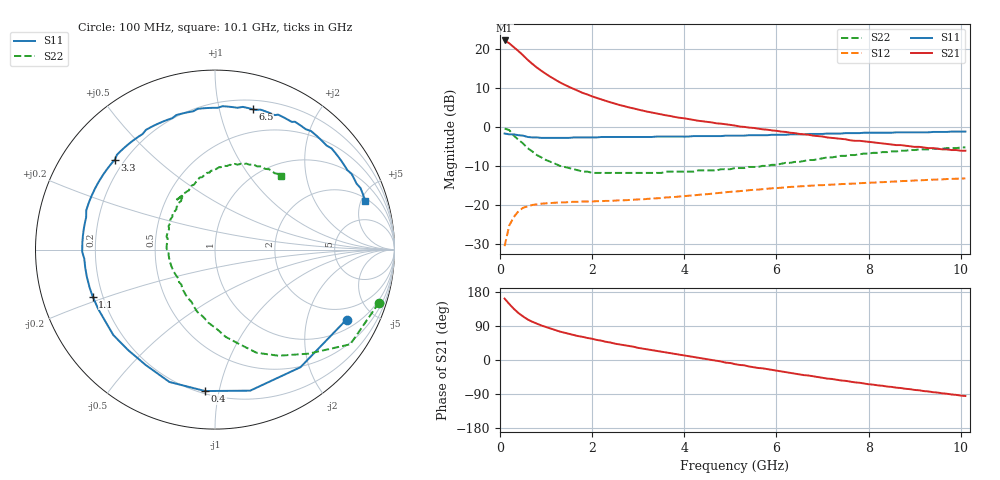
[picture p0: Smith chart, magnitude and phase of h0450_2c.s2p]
!HBFP-0450
!S and NOISE PARAMETERS at Vce=2V  Ic=5mA.  LAST UPDATED  09-04-98
# GHZ S MA R  50
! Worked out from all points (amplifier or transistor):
!   101 points, 100 MHz to 10.1 GHz, reference 50 ohm
!   highest |S21| = 22.2 dB at 100 MHz (marker M1)
!   |S21| within 3 dB of that: start of sweep to 426.5 MHz
!   unconditionally stable (mu >= 1): 2.927 GHz to end of sweep
!   at 1.7 GHz: K = 0.62, MSG = 14.2 dB, |S12| = -19.1 dB
!   at 5.1 GHz: K = 1.22, MAG = 5.6 dB, |S12| = -16.5 dB
!   at 10.1 GHz: K = 1.09, MAG = 1.7 dB, |S12| = -13.1 dB
!   lowest NFmin = 1.21 dB at 1.8 GHz
!   S11 on the Smith chart (normalised r, x): 100 MHz: 1.39, -3.49; 400 MHz: 0.22, -0.91; 1.1 GHz: 0.16, -0.18; 3.3 GHz: 0.16, +0.37; 6.5 GHz: 0.28, +1.27; 10.1 GHz: 2.24, +5.41
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0.1  0.83 -28.0  12.9 162.0  0.03 75.0  0.96 -18.0
0.2  0.81 -54.0  11.87 148.0  0.055 61.0  0.92 -35.0
0.3  0.81 -76.0  10.57 135.0  0.071 51.0  0.78 -48.0
0.4  0.79 -94.0  9.44 124.0  0.084 42.0  0.69 -59.0
0.5  0.78 -109.0  8.33 115.0  0.093 35.0  0.62 -68.0
0.6  0.75 -121.0  7.29 107.0  0.097 30.0  0.54 -76.0
0.7  0.74 -131.0  6.48 101.0  0.101 26.0  0.49 -83.0
0.9  0.73 -147.0  5.26 91.0  0.105 20.0  0.41 -95.0
1.1  0.73 -159.0  4.4 83.0  0.107 16.0  0.36 -106.0
1.3  0.73 -168.0  3.75 75.0  0.109 13.0  0.32 -114.0
1.6  0.74 -179.0  3.09 66.0  0.111 10.0  0.29 -127.0
1.8  0.74 174.0  2.74 61.0  0.112 8.0  0.27 -134.0
2.1  0.74 166.0  2.37 53.0  0.113 6.0  0.26 -145.0
2.5  0.75 156.0  2 43.0  0.115 4.0  0.26 -156.0
3.3  0.75 138.0  1.54 26.0  0.122 2.0  0.26 -175.0
3.5  0.76 134.0  1.46 22.0  0.124 1.0  0.26 -179.0
5.1  0.78 102.0  1.05 -11.0  0.15 -9.0  0.3 146.0
6.3  0.81 79.0  0.85 -34.0  0.172 -20.0  0.35 129.0
6.5  0.81 75.0  0.82 -38.0  0.175 -23.0  0.36 114.0
6.8  0.82 70.0  0.78 -43.0  0.179 -26.0  0.38 108.0
8.5  0.85 43.0  0.6 -71.0  0.201 -45.0  0.49 77.0
10.1  0.88 18.0  0.5 -95.0  0.221 -67.0  0.55 48.0
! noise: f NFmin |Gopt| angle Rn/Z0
1.8  1.21  0.53  163  0.04
2  1.27  0.52  171  0.05
2.5  1.44  0.58  -171  0.05
3.5  1.77  0.66  -144  0.15
4  1.94  0.68  -131  0.27
5  2.27  0.74  -109  0.67
5.5  2.5  0.77  -98  0.99
7  2.94  0.82  -68  2.43
8  3.27  0.84  -50  3.81
10  3.94  0.84  -20  6.56
